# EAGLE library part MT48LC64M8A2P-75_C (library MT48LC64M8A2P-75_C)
DRAM 512Mb, 3.3v, 133Mhz 64M x 8 SDR Source: Datasheet
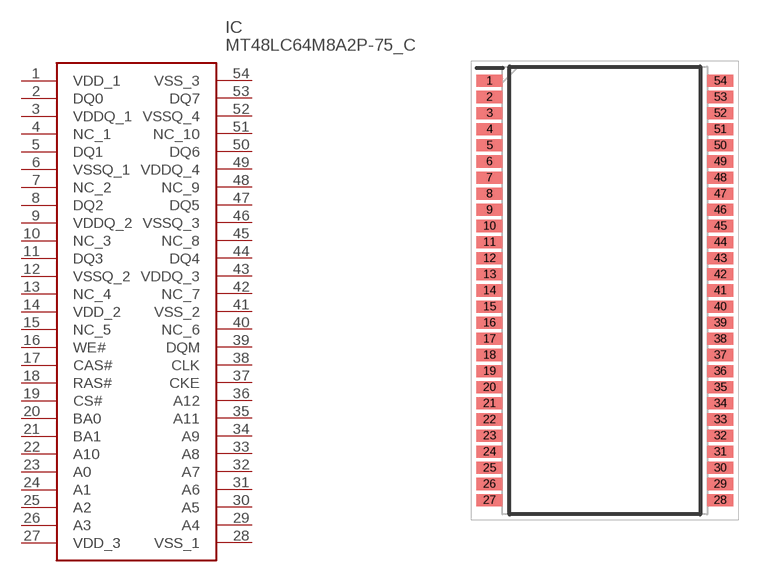
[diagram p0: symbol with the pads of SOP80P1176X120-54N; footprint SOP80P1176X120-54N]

Designator prefix IC

## MT48LC64M8A2P-75_C (Description: DRAM 512Mb, 3.3v, 133Mhz 64M x 8 SDR; Height: 1.2mm; Manufacturer_Name: Alliance Memory; Manufacturer_Part_Number: MT48LC64M8A2P-75:C; Mouser_Part_Number: 913-MT48LC64M8A2P75C; Mouser_Price-Stock: https://www.mouser.com/Search/Refine.aspx?Keyword=913-MT48LC64M8A2P75C)  [SOP80P1176X120-54N]
1  VDD_1
2  DQ0
3  VDDQ_1
4  NC_1
5  DQ1
6  VSSQ_1
7  NC_2
8  DQ2
9  VDDQ_2
10  NC_3
11  DQ3
12  VSSQ_2
13  NC_4
14  VDD_2
15  NC_5
16  WE#
17  CAS#
18  RAS#
19  CS#
20  BA0
21  BA1
22  A10
23  A0
24  A1
25  A2
26  A3
27  VDD_3
28  VSS_1
29  A4
30  A5
31  A6
32  A7
33  A8
34  A9
35  A11
36  A12
37  CKE
38  CLK
39  DQM
40  NC_6
41  VSS_2
42  NC_7
43  VDDQ_3
44  DQ4
45  NC_8
46  VSSQ_3
47  DQ5
48  NC_9
49  VDDQ_4
50  DQ6
51  NC_10
52  VSSQ_4
53  DQ7
54  VSS_3

## Footprint SOP80P1176X120-54N (pad centres in mm)
54 Pin TSSOP II (400 mil) TG/P PACKAGE
smd 1.295 x 0.6: 1 -5.728,10.4; 2 -5.728,9.6; 3 -5.728,8.8; 4 -5.728,8; 5 -5.728,7.2; 6 -5.728,6.4; 7 -5.728,5.6; 8 -5.728,4.8; 9 -5.728,4; 10 -5.728,3.2; 11 -5.728,2.4; 12 -5.728,1.6; 13 -5.728,0.8; 14 -5.728,0; 15 -5.728,-0.8; 16 -5.728,-1.6; 17 -5.728,-2.4; 18 -5.728,-3.2; 19 -5.728,-4; 20 -5.728,-4.8; 21 -5.728,-5.6; 22 -5.728,-6.4; 23 -5.728,-7.2; 24 -5.728,-8; 25 -5.728,-8.8; 26 -5.728,-9.6; 27 -5.728,-10.4; 28 5.728,-10.4; 29 5.728,-9.6; 30 5.728,-8.8; 31 5.728,-8; 32 5.728,-7.2; 33 5.728,-6.4; 34 5.728,-5.6; 35 5.728,-4.8; 36 5.728,-4; 37 5.728,-3.2; 38 5.728,-2.4; 39 5.728,-1.6; 40 5.728,-0.8; 41 5.728,0; 42 5.728,0.8; 43 5.728,1.6; 44 5.728,2.4; 45 5.728,3.2; 46 5.728,4; 47 5.728,4.8; 48 5.728,5.6; 49 5.728,6.4; 50 5.728,7.2; 51 5.728,8; 52 5.728,8.8; 53 5.728,9.6; 54 5.728,10.4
